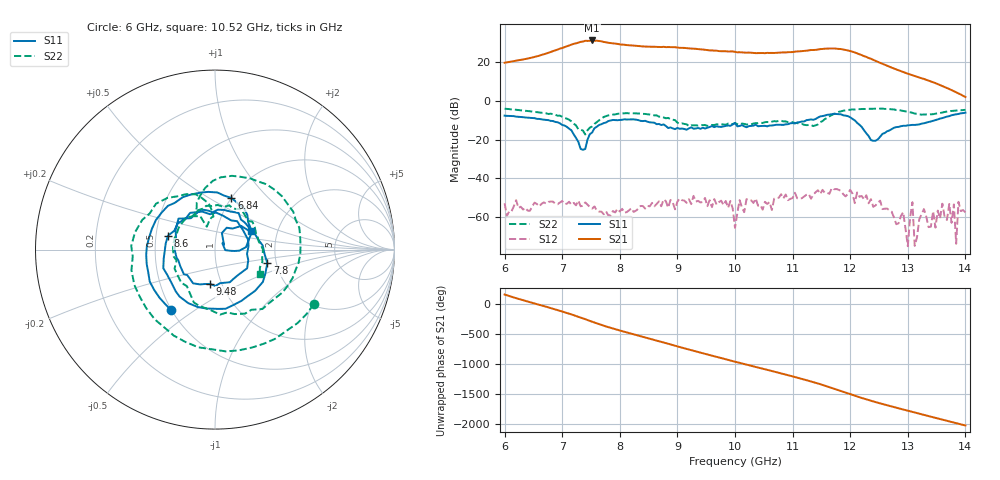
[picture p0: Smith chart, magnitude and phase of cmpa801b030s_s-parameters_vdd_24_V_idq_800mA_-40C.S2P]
!Keysight Technologies,E5071C,MY46110325,B.14.03
!Date: Tue Aug 11 10:47:02 2020
!Data & Calibration Information:
!Freq	S11:SOLT2(ON)	S21:SOLT2(ON)	S12:SOLT2(ON)	S22:SOLT2(ON)
!PortZ  Port1:50+j0  Port2:50+j0
!Above PortZ is port z conversion or system Z0 setting when saving the data.
!When reading, reference impedance value at option line is always used.
# Hz S dB R 50
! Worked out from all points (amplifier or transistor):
!   201 points, 6 GHz to 14 GHz, reference 50 ohm
!   highest |S21| = 31.4 dB at 7.52 GHz (marker M1)
!   |S21| within 3 dB of that: 7.081 GHz to 8.368 GHz (1.288 GHz wide, 16.7 % of centre)
!   unconditionally stable (mu >= 1): start of sweep to end of sweep
!   at 7.32 GHz: K = 7.61, MAG = 30.8 dB, |S12| = -54.6 dB
!   at 10 GHz: K = 44.76, MAG = 26.1 dB, |S12| = -65.8 dB
!   at 14 GHz: K = 149.34, MAG = 5.1 dB, |S12| = -57.7 dB
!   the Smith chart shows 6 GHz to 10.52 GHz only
!   S11 on the Smith chart (normalised r, x): 6 GHz: 0.50, -0.40; 6.84 GHz: 1.00, +0.63; 7.8 GHz: 1.79, -0.30; 8.6 GHz: 0.58, +0.10; 9.48 GHz: 0.88, -0.35; 10.52 GHz: 1.46, +0.32
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6e9  -7.61 -126.4  19.80 160.3  -53.03 -54.2  -4.02 -29.0
6.36e9  -8.56 169.4  21.73 54.6  -55.38 -148.7  -5.11 -92.1
6.84e9  -10.41 72.4  25.81 -75.3  -52.16 124.2  -6.82 167.8
7.2e9  -17.31 -2.5  29.62 176.1  -52.84 33.3  -11.74 97.6
7.36e9  -25.30 40.9  30.78 122.7  -54.30 -14.7  -15.37 99.9
7.52e9  -16.34 50.2  31.36 67.7  -55.80 -57.7  -13.22 121.6
7.8e9  -10.42 -14.7  30.16 -21.8  -59.26 -170.6  -7.50 77.0
8.08e9  -9.50 -80.0  29.15 -99.4  -57.95 82.4  -6.41 31.8
8.32e9  -9.92 -133.3  28.48 -163.3  -55.88 21.7  -6.45 -2.9
8.6e9  -11.27 163.6  28.10 123.5  -54.60 -34.6  -7.47 -45.3
8.68e9  -11.92 144.5  28.01 102.4  -52.03 -79.7  -8.13 -58.8
9.08e9  -14.30 16.6  27.54 -3.4  -51.43 -173.5  -11.59 -135.5
9.48e9  -14.29 -98.0  26.51 -108.4  -50.29 84.0  -12.48 131.1
1e10  -11.48 139.7  25.49 121.5  -65.80 -88.9  -11.42 56.9
1.052e10  -12.89 27.0  24.76 -3.3  -52.29 -154.4  -10.97 -28.3
1.092e10  -12.03 -45.2  25.29 -102.4  -51.41 90.5  -10.97 -83.4
1.136e10  -9.76 -124.2  26.41 141.1  -48.57 8.2  -13.02 160.3
1.156e10  -7.56 -160.6  27.09 83.5  -47.64 -71.2  -9.37 96.9
1.18e10  -6.82 144.6  26.98 6.9  -46.05 -135.8  -5.64 27.6
1.208e10  -10.06 76.0  25.15 -83.7  -52.96 150.6  -4.45 -45.1
1.268e10  -15.29 178.9  17.75 106.5  -56.68 -34.7  -4.22 -160.0
1.4e10  -6.06 -134.2  2.04 140.8  -57.71 114.4  -4.61 -48.3
